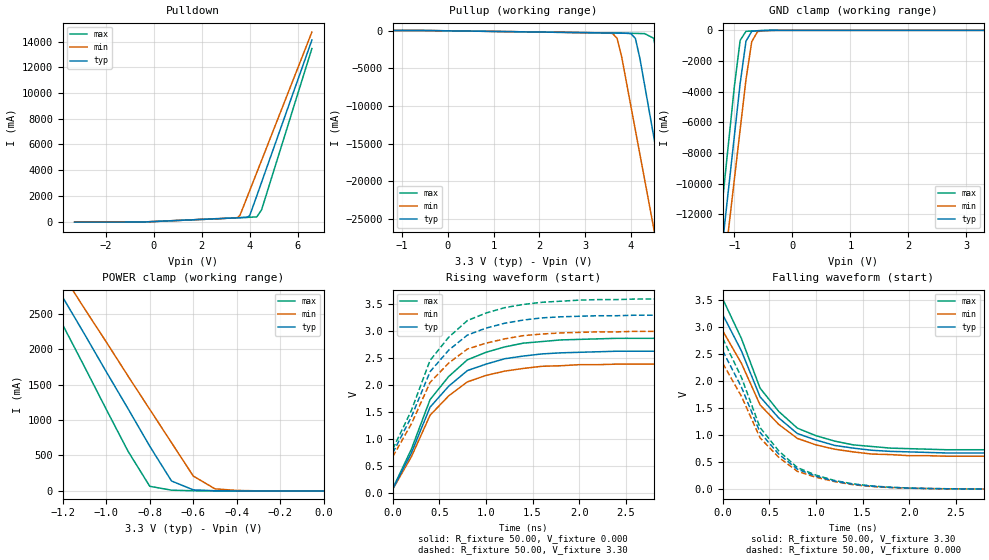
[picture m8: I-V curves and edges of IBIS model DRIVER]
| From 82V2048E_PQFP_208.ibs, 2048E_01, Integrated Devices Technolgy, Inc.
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|   Model DRIVER
[Model]   DRIVER
Model_type   3-state
Polarity   Non-Inverting
Enable   Active-Low
C_comp   40.00pF   NA   NA
[Temperature Range]   25.00   85.00   -40.00
[Voltage Range]   3.30V   3.00V   3.60V
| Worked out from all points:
|   slope of the pulldown table from 0 to 0.495 V, typ, clamps not added: 12.1 ohm
|   slope of the pullup table from 0 to 0.495 V, typ, clamps not added: 12.3 ohm
|   GND clamp passes 1 mA (typ) near -0.32 V on its own axis
|   POWER clamp passes 1 mA (typ) near -0.44 V on its own axis
|   rising waveform, R_fixture 50.00, V_fixture 0.000: 20-80 % time 542ps typ, 542ps min, 545ps max; typ from 0.072 V to 2.63 V
|   rising waveform, R_fixture 50.00, V_fixture 3.30: 20-80 % time 546ps typ, 543ps min, 543ps max; typ from 0.74 V to 3.3 V
|   falling waveform, R_fixture 50.00, V_fixture 3.30: 20-80 % time 542ps typ, 542ps min, 545ps max; typ from 3.23 V to 0.67 V
|   falling waveform, R_fixture 50.00, V_fixture 0.000: 20-80 % time 546ps typ, 543ps min, 543ps max; typ from 2.56 V to 0 V
[Pulldown]
| voltage   I(typ)   I(min)   I(max)
-3.3V     -46.68mA   -33.31mA   -51.6mA
-300mV    -25.11mA   -23.01mA   -25.29mA
3.5V      290mA      310mA      290mA
3.6V      300mA      490mA      300mA
3.9V      330mA      1.91A      320mA
4V        450mA      2.38A      330mA
4.3V      2A         3.81A      360mA
4.5V      3.05A      4.75A      910mA
6.6V      14.12A     14.74A     13.46A
[Pullup]
| voltage   I(typ)   I(min)   I(max)
-3.3V     47.12mA    34.18mA    62.58mA
3.6V      -290mA     -350mA     -290mA
3.7V      -300mA     -1A        -300mA
3.8V      -320mA     -3.48A     -310mA
4.1V      -1.02A     -13.24A    -340mA
4.3V      -7.19A     -19.74A    -370mA
4.5V      -14.06A    -26.25A    -990mA
4.7V      -20.93A    -32.76A    -7.64A
4.9V      -27.8A     -39.26A    -14.96A
5.1V      -34.67A    -45.77A    -22.27A
5.3V      -41.54A    -52.27A    -29.58A
6.6V      -86.2A     -94.56A    -77.12A
[GND_clamp]
| voltage   I(typ)   I(min)   I(max)
-3.3V     -85.89A    -84.53A    -87.75A
-1.3V     -17.18A    -19.47A    -14.62A
-1.2V     -13.75A    -16.22A    -10.97A
-1.1V     -10.32A    -12.97A    -7.31A
-1V       -6.88A     -9.71A     -3.65A
-900mV    -3.45A     -6.46A     -650mA
-800mV    -710mA     -3.21A     -66.68mA
-700mV    -63.03mA   -730mA     -41.83mA
-600mV    -26.66mA   -81.9mA    -26.86mA
-200mV    -12.87uA   -290uA     -1.95uA
3.3V      21.15nA    540uA      650pA
[POWER_clamp]
| voltage   I(typ)   I(min)   I(max)
-3.3V     13.8A      13.02A     14.9A
-1.3V     3.26A      3.52A      2.94A
-1.2V     2.73A      3.05A      2.34A
-1.1V     2.21A      2.57A      1.75A
-900mV    1.16A      1.62A      560mA
-800mV    630mA      1.15A      65.09mA
-700mV    140mA      680mA      10.65mA
-600mV    15.15mA    210mA      2.26mA
-500mV    2.56mA     29.16mA    150uA
-300mV    4.14uA     900uA      120nA
0V        4.17nA     950nA      79.6pA
[Ramp]
| variable   typ   min   max
dV/dt_r   1.58/0.56n   1.44/0.56n   1.72/0.56n
dV/dt_f   1.58/0.56n   1.44/0.56n   1.72/0.56n
R_load = 50.00
[Rising Waveform]
R_fixture = 50.00
V_fixture = 0.000
V_fixture_min = 0.000
V_fixture_max = 0.000
| time   V(typ)   V(min)   V(max)
0s        71.76mV    65.24mV    78.28mV
200ps     740mV      670mV      810mV
400ps     1.59V      1.44V      1.73V
600ps     1.98V      1.8V       2.16V
800ps     2.27V      2.06V      2.47V
1.2ns     2.49V      2.26V      2.71V
1.4ns     2.54V      2.31V      2.78V
1.6ns     2.58V      2.35V      2.81V
2.4ns     2.63V      2.39V      2.87V
10ns      2.63V      2.39V      2.87V
[Rising Waveform]
R_fixture = 50.00
V_fixture = 3.30
V_fixture_min = 3.00
V_fixture_max = 3.60
| time   V(typ)   V(min)   V(max)
0s        740mV      670mV      810mV
200ps     1.41V      1.28V      1.53V
400ps     2.25V      2.05V      2.46V
600ps     2.65V      2.41V      2.89V
800ps     2.93V      2.67V      3.2V
1.2ns     3.15V      2.86V      3.44V
1.4ns     3.21V      2.92V      3.5V
1.8ns     3.27V      2.97V      3.56V
2.6ns     3.3V       3V         3.6V
10ns      3.3V       3V         3.6V
[Falling Waveform]
R_fixture = 50.00
V_fixture = 3.30
V_fixture_min = 3.00
V_fixture_max = 3.60
| time   V(typ)   V(min)   V(max)
0s        3.23V      2.93V      3.52V
200ps     2.56V      2.33V      2.79V
400ps     1.71V      1.56V      1.87V
600ps     1.32V      1.2V       1.44V
800ps     1.03V      940mV      1.13V
1.2ns     810mV      740mV      890mV
1.4ns     760mV      690mV      820mV
1.8ns     700mV      640mV      760mV
2.4ns     670mV      610mV      730mV
10ns      670mV      610mV      730mV
[Falling Waveform]
R_fixture = 50.00
V_fixture = 0.000
V_fixture_min = 0.000
V_fixture_max = 0.000
| time   V(typ)   V(min)   V(max)
0s        2.56V      2.33V      2.79V
200ps     1.89V      1.72V      2.07V
400ps     1.05V      950mV      1.14V
600ps     650mV      590mV      710mV
800ps     370mV      330mV      400mV
1ns       240mV      220mV      260mV
1.4ns     89.64mV    81.49mV    97.79mV
1.8ns     32.6mV     29.63mV    35.56mV
2.6ns     4.31mV     3.92mV     4.7mV
10ns      32.35pV    29.41pV    35.29pV
